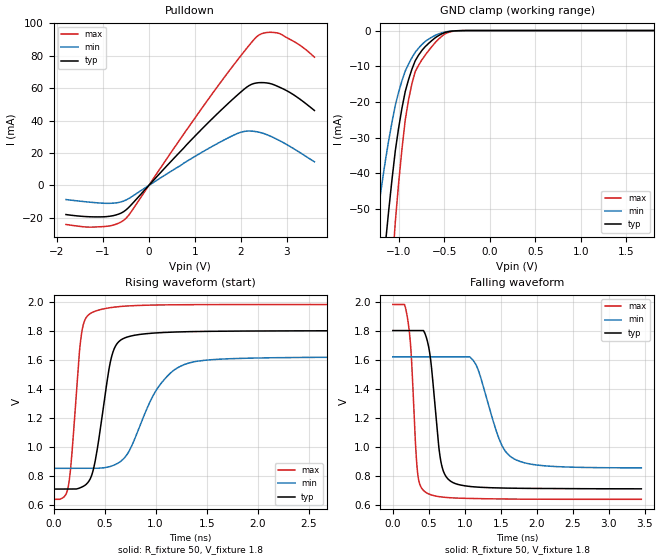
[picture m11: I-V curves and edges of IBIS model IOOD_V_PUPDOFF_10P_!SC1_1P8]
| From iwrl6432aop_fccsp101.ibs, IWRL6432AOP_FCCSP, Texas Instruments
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|   Model Cell IOOD_V_PUPDOFF_10P_!SC1_1P8
|IOOD_V_PUPDOFF_10P_!SC1_1P8
[Model]   IOOD_V_PUPDOFF_10P_!SC1_1P8
Model_type   I/O_open_drain
Polarity   Non-Inverting
Enable   Active-Low
Vinl =  0.63
Vinh =  1.17
Cref =  15pF
Rref =  100.0000M
Vref =  0V
Vmeas =  0.9
|   typ   min   max
C_comp   2.290246p   2.205796p   2.292736p
[Model Spec]
Vinl   0.63   0.567   0.693
Vinh   1.17   1.053   1.287
[Temperature Range]   25   125   -40
[Voltage Range]   1.8   1.62   1.98
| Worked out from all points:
|   slope of the pulldown table from 0 to 0.27 V, typ, clamps not added: 32.2 ohm
|   GND clamp passes 1 mA (typ) near -0.53 V on its own axis
|   rising waveform, R_fixture 50, V_fixture 1.8: 20-80 % time 141ps typ, 321ps min, 87.5ps max; typ from 0.709 V to 1.8 V
|   falling waveform, R_fixture 50, V_fixture 1.8: 20-80 % time 128ps typ, 290ps min, 84.1ps max; typ from 1.8 V to 0.71 V
| Where Nom  PVT is Nominal Process, 1.8V, 25C
|   Fast PVT is Strong Process,  1.98V, -40C
|   Slow PVT is Weak Process,   1.62V, 125C
[Pulldown]
|   voltage   I(typ)   I(min)   I(max)
-1.8V     -17.92mA   -8.674mA   -24.03mA
-927.3mV  -19.22mA   -10.99mA   -25.2mA
-654.5mV  -17.65mA   -10.46mA   -23.22mA
-490.9mV  -14.97mA   -8.904mA   -20.12mA
872.7mV   26.63mA    15.72mA    36.29mA
1.691V    49.7mA     28.87mA    68.59mA
2.127V    60.63mA    33.53mA    84.59mA
2.4V      63.43mA    32.84mA    92.9mA
2.618V    62.99mA    30.74mA    94.47mA
2.836V    60.69mA    27.76mA    93.76mA
3.273V    53.49mA    20.53mA    86.73mA
3.6V      46.26mA    14.64mA    79.11mA
[GND_clamp]
|   voltage   I(typ)   I(min)   I(max)
-1.8V     -270.2mA   -170.2mA   -430.1mA
-1.255V   -91.66mA   -55.91mA   -148.4mA
-1.145V   -59.91mA   -36.44mA   -97.09mA
-1.109V   -50.48mA   -30.83mA   -81.55mA
-1.073V   -41.73mA   -25.65mA   -67.05mA
-1.036V   -33.66mA   -20.92mA   -53.59mA
-927.3mV  -17.07mA   -11.35mA   -25.04mA
-854.5mV  -10.86mA   -7.616mA   -14.91mA
-781.8mV  -6.919mA   -4.945mA   -9.771mA
-636.4mV  -2.823mA   -1.868mA   -4.529mA
-381.8mV  -84.73uA   -78.7uA    -126.1uA
1.8V      19.3nA     3.129uA    310.3nA
[Ramp]
| variable   typ   min   max
dV/dt_f 0.66582244/0.13064135n 0.47095698/0.29741514n 0.81505832/85.878667p
dV/dt_r 0.66457081/0.1768972n 0.48134805/0.39636116n 0.81913391/99.774546p
R_load = 50
[Rising Waveform]
R_fixture = 50
V_fixture = 1.8
V_fixture_min = 1.62
V_fixture_max = 1.98
|   time   V(typ)   V(min)   V(max)
0s        709.4mV    852.1mV    638.8mV
143.7ps   709.4mV    852.1mV    723.5mV
176.4ps   709.4mV    852.1mV    921.3mV
269.4ps   720.7mV    852.1mV    1.755V
369.4ps   795.8mV    852.1mV    1.922V
561.6ps   1.6V       866.3mV    1.959V
688.2ps   1.747V     919.4mV    1.968V
1.012ns   1.785V     1.396V     1.977V
1.287ns   1.792V     1.568V     1.979V
3.453ns   1.8V       1.618V     1.98V
[Falling Waveform]
R_fixture = 50
V_fixture = 1.8
V_fixture_min = 1.62
V_fixture_max = 1.98
|   time   V(typ)   V(min)   V(max)
0s        1.8V       1.619V     1.979V
200.1ps   1.8V       1.619V     1.897V
252.3ps   1.8V       1.619V     1.661V
340ps     1.8V       1.619V     840.9mV
445.1ps   1.782V     1.619V     690.7mV
662ps     914.5mV    1.619V     655mV
801.1ps   763.4mV    1.619V     648.7mV
1.144ns   723.3mV    1.575V     643.6mV
1.675ns   714.4mV    919.6mV    639.5mV
3.453ns   710.3mV    854.5mV    638mV
